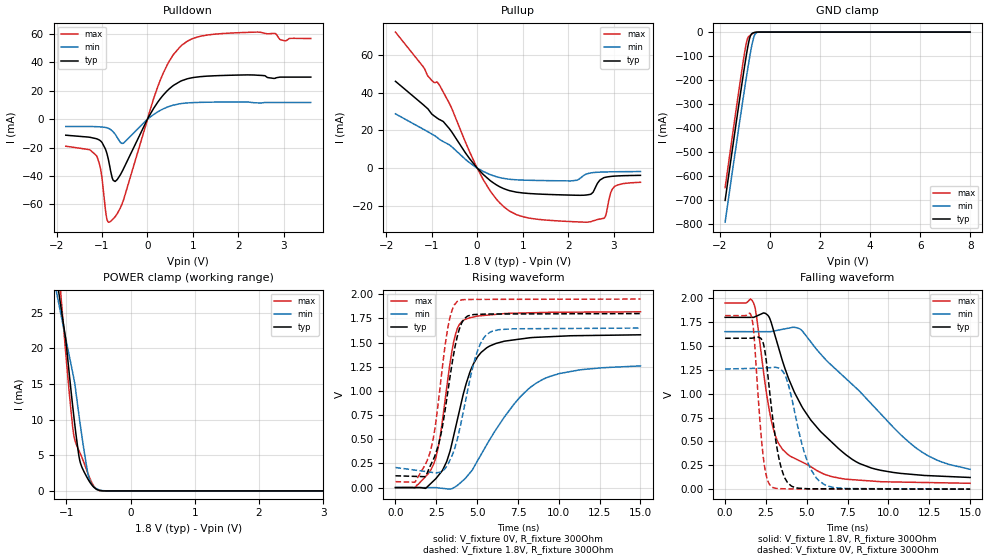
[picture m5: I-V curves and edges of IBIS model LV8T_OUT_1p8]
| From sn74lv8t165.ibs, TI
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[Model]   LV8T_OUT_1p8
Model_type   3-state
Polarity   Non-Inverting
Enable   Active-Low
Vmeas = 0.9
Vref = 0
Cref = 15pF
Rref = 1000
|   typ   min   max
C_comp   1.25pF   1.25pF   1.25pF
[Voltage Range]   1.8   1.65   1.95
[Temperature Range]   27   125   -40
[Pullup Reference]   1.8   1.65   1.95
[Pulldown Reference]   0   0   0
[Power Clamp Reference]   1.8   1.65   1.95
[GND Clamp Reference]   0   0   0
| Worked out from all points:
|   slope of the pulldown table from 0 to 0.27 V, typ, clamps not added: 19.4 ohm
|   slope of the pullup table from 0 to 0.27 V, typ, clamps not added: 42.7 ohm
|   GND clamp passes 1 mA (typ) near -0.60 V on its own axis
|   POWER clamp passes 1 mA (typ) near -0.62 V on its own axis
|   falling waveform, V_fixture 1.8V, R_fixture 300Ohm: 20-80 % time 3.44ns typ, 5.1ns min, 1.32ns max; typ from 1.8 V to 0.122 V
|   rising waveform, V_fixture 0V, R_fixture 300Ohm: 20-80 % time 1.51ns typ, 3.12ns min, 956ps max; typ from 0 V to 1.58 V
|   rising waveform, V_fixture 1.8V, R_fixture 300Ohm: 20-80 % time 999ps typ, 1.15ns min, 903ps max; typ from 0.122 V to 1.8 V
|   falling waveform, V_fixture 0V, R_fixture 300Ohm: 20-80 % time 730ps typ, 1.13ns min, 485ps max; typ from 1.58 V to 0 V
[Pulldown]
|   Voltage   I(typ)   I(min)   I(max)
-1.796V   -11.28mA   -5.119mA   -19.02mA
-1.125V   -13.75mA   -5.279mA   -25.54mA
-1.02V    -15.68mA   -5.488mA   -37.25mA
-893.5mV  -24.03mA   -6.033mA   -70.1mA
-830.5mV  -33.05mA   -6.918mA   -72.34mA
-757mV    -42.89mA   -8.838mA   -70.24mA
-662.5mV  -42.35mA   -13.04mA   -66.33mA
-526mV    -34.77mA   -16.86mA   -56.7mA
230mV     12.16mA    5.227mA    23.22mA
723.5mV   26.62mA    10.88mA    51.12mA
1.752V    30.81mA    12.08mA    60.4mA
3.59V     29.56mA    11.75mA    56.71mA
[GND Clamp]
|   Voltage   I(typ)   I(min)   I(max)
-1.796V   -700.9mA   -791.6mA   -647.7mA
-1.219V   -281.3mA   -376.1mA   -223.6mA
-1.051V   -164.4mA   -259.1mA   -107.3mA
-956.5mV  -102mA     -195.1mA   -50.21mA
-883mV    -57.78mA   -146.8mA   -23.05mA
-788.5mV  -16.94mA   -88.19mA   -12.93mA
-736mV    -7.235mA   -59.04mA   -9.144mA
-673mV    -3.075mA   -29.92mA   -5.317mA
-631mV    -1.745mA   -15.92mA   -3.28mA
-568mV    -592.8uA   -4.575mA   -1.137mA
-421mV    -9.243uA   -103.9uA   -7.132uA
8V        0A         0A         0A
[Pullup]
|   Voltage   I(typ)   I(min)   I(max)
-1.796V   46.04mA    28.76mA    72.15mA
-1.093V   31.62mA    19.36mA    49.12mA
-830.5mV  25.7mA     15.25mA    44.09mA
135.5mV   -3.465mA   -1.843mA   -6.241mA
429.5mV   -9.049mA   -4.663mA   -16.7mA
723.5mV   -12.09mA   -5.999mA   -23.02mA
2.067V    -14.39mA   -6.831mA   -28.44mA
2.487V    -13.97mA   -2.616mA   -28.53mA
2.803V    -5.024mA   -2.093mA   -26.34mA
2.929V    -4.496mA   -2.022mA   -13.69mA
3.013V    -4.313mA   -1.988mA   -9.947mA
3.59V     -3.9mA     -1.879mA   -7.587mA
[POWER Clamp]
|   Voltage   I(typ)   I(min)   I(max)
-1.796V   71.37mA    58.65mA    87.68mA
-1.135V   28.87mA    27.05mA    31.94mA
-1.103V   26.96mA    25.62mA    29.38mA
-1.083V   25.68mA    24.67mA    27.18mA
-1.009V   21.17mA    21.37mA    19.28mA
-925mV    13.88mA    17.64mA    11.01mA
-883mV    10.43mA    15.76mA    7.781mA
-788.5mV  4.183mA    9.633mA    5.343mA
-662.5mV  1.647mA    2.362mA    2.407mA
-589mV    682.9uA    753.1uA    922.8uA
-484mV    68.78uA    128.6uA    47.06uA
8V        0A         0A         0A
[Ramp]
R_load = 300
|   typ   min   max
dV/dt_r   0.94808/1.49763e-09   0.754867/3.09883e-09   1.09079/9.51431e-10
dV/dt_f   1.00648/3.43435e-09   0.865073/5.09841e-09   1.13295/1.31216e-09
[Falling Waveform]
V_fixture = 1.8V
V_fixture_min = 1.65V
V_fixture_max = 1.95V
R_fixture = 300Ohm
C_fixture = 0F
|   Time   V(typ)   V(min)   V(max)
0s        1.8V       1.65V      1.95V
1.751ns   1.8V       1.65V      1.948V
2.474ns   1.84V      1.65V      1.075V
2.863ns   1.722V     1.652V     693.4mV
3.264ns   1.487V     1.666V     482.6mV
3.866ns   1.167V     1.686V     360.1mV
5.248ns   723.1mV    1.542V     234.7mV
7.999ns   289.3mV    1.063V     97mV
11.81ns   149.4mV    417mV      71.16mV
15ns      122.4mV    208.2mV    61.71mV
[Rising Waveform]
V_fixture = 0V
V_fixture_min = 0V
V_fixture_max = 0V
R_fixture = 300Ohm
C_fixture = 0F
|   Time   V(typ)   V(min)   V(max)
0s        188.7uV    543.5uV    79.57uV
1.188ns   545.1uV    408.6uV    -4.702mV
2.334ns   70.1mV     278.5uV    241.7mV
2.73ns    146.3mV    -4.788mV   523mV
3.545ns   522mV      -4.28mV    1.491V
4.099ns   928.5mV    67.78mV    1.723V
4.788ns   1.284V     206.8mV    1.765V
5.583ns   1.446V     442.6mV    1.783V
8.617ns   1.554V     1.081V     1.809V
15ns      1.58V      1.259V     1.818V
[Rising Waveform]
V_fixture = 1.8V
V_fixture_min = 1.65V
V_fixture_max = 1.95V
R_fixture = 300Ohm
C_fixture = 0F
|   Time   V(typ)   V(min)   V(max)
0s        122.4mV    208.2mV    61.71mV
1.188ns   116.3mV    181.2mV    55.95mV
2.055ns   197.3mV    161.5mV    330.4mV
2.713ns   495.7mV    159.7mV    1.01V
3.207ns   992.1mV    241.7mV    1.651V
3.782ns   1.561V     498.3mV    1.926V
4.209ns   1.744V     828.9mV    1.944V
4.962ns   1.791V     1.383V     1.947V
5.772ns   1.795V     1.605V     1.947V
15ns      1.8V       1.65V      1.95V
[Falling Waveform]
|Gnd
V_fixture = 0V
V_fixture_min = 0V
V_fixture_max = 0V
R_fixture = 300Ohm
C_fixture = 0F
|   Time   V(typ)   V(min)   V(max)
0s        1.58V      1.259V     1.818V
1.612ns   1.581V     1.265V     1.809V
1.762ns   1.585V     1.265V     1.628V
2.334ns   1.529V     1.268V     340.9mV
2.863ns   814.3mV    1.274V     22.92mV
3.34ns    287.6mV    1.262V     5.814mV
3.817ns   69.98mV    1.125V     3.134mV
5.002ns   5.315mV    307.6mV    2.81mV
6.1ns     3.706mV    46.02mV    2.51mV
15ns      188.7uV    543.3uV    79.57uV
